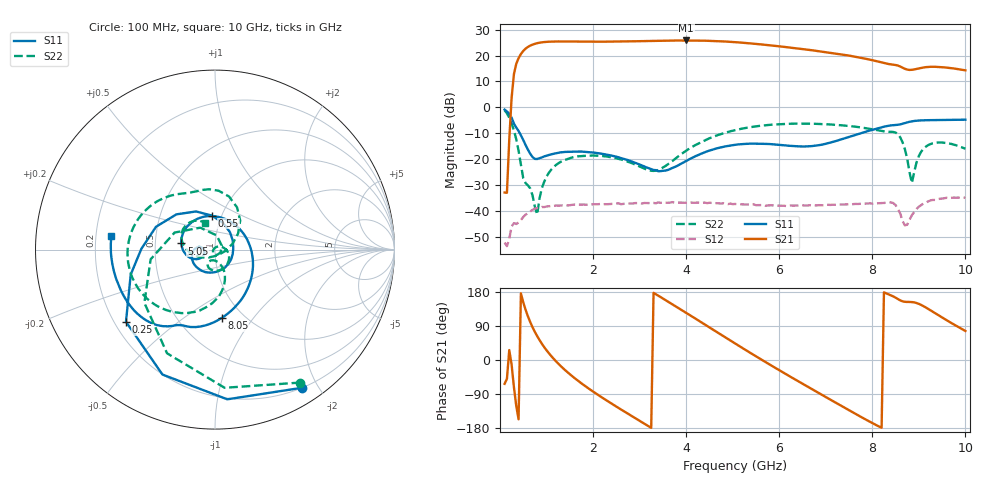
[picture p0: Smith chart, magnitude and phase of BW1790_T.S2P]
!Keysight Technologies,N5245A,MY52451660,A.10.49.11
!Date: Monday, August 07, 2017 16:27:22
!Correction: S11(Full 2 Port(1,2))
!S21(Full 2 Port(1,2))
!S12(Full 2 Port(1,2))
!S22(Full 2 Port(1,2))
!S2P File: Measurements: S11, S21, S12, S22:
# Hz S  dB  R 50
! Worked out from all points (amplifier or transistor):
!   199 points, 100 MHz to 10 GHz, reference 50 ohm
!   highest |S21| = 25.8 dB at 4 GHz (marker M1)
!   |S21| within 3 dB of that: 562.9 MHz to 6.354 GHz (5.791 GHz wide, 167 % of centre)
!   unconditionally stable (mu >= 1): start of sweep to end of sweep
!   at 1.75 GHz: K = 2.08, MAG = 25.5 dB, |S12| = -37.4 dB
!   at 5.05 GHz: K = 1.85, MAG = 25.8 dB, |S12| = -37.1 dB
!   at 10 GHz: K = 3.53, MAG = 16.1 dB, |S12| = -34.8 dB
!   S11 on the Smith chart (normalised r, x): 100 MHz: 0.20, -1.79; 250 MHz: 0.25, -0.34; 550 MHz: 0.90, +0.35; 5.05 GHz: 0.68, +0.05; 8.05 GHz: 0.80, -0.71; 10 GHz: 0.27, +0.06
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1e8  -0.82 -57.8  -32.75 -62.9  -51.98 17.9  -1.11 -57.3
2.5e8  -3.90 -141.0  3.56 -11.9  -45.81 -12.4  -6.15 -143.0
3e8  -6.20 -163.5  12.81 -71.2  -44.54 -48.9  -8.81 -171.4
3.5e8  -7.75 179.2  16.79 -121.0  -44.85 -87.8  -12.24 157.1
4.5e8  -10.71 137.6  20.58 175.8  -43.36 -169.7  -22.00 83.1
5.5e8  -14.43 95.0  22.63 132.8  -41.27 133.9  -29.10 -28.3
7.5e8  -19.81 4.9  24.50 74.2  -38.97 76.0  -38.24 -158.8
1.05e9  -18.30 -80.9  25.32 18.0  -38.02 33.0  -25.18 6.2
1.35e9  -17.22 -118.4  25.41 -21.2  -37.67 7.9  -20.53 -33.9
1.75e9  -16.98 -148.4  25.34 -61.6  -37.42 -14.0  -18.73 -69.5
2.45e9  -18.74 179.9  25.36 -119.1  -37.07 -47.2  -19.34 -108.6
2.95e9  -21.59 170.5  25.51 -156.7  -36.81 -66.4  -22.37 -117.5
3.4e9  -24.56 -175.4  25.67 169.9  -36.55 -83.9  -24.08 -86.7
4e9  -20.61 -149.6  25.80 124.5  -36.69 -109.5  -16.65 -68.3
4.5e9  -16.61 -162.4  25.65 86.1  -36.69 -127.8  -11.86 -84.3
5.05e9  -14.38 169.6  25.14 43.7  -37.14 -147.6  -8.71 -108.5
5.75e9  -14.04 123.2  24.02 -8.7  -37.72 -169.7  -6.76 -140.2
6.7e9  -14.87 33.3  22.04 -76.7  -37.72 163.3  -6.25 -179.4
7.45e9  -11.62 -40.9  20.11 -129.1  -37.30 138.4  -7.04 150.6
8.05e9  -8.35 -84.3  18.00 -169.7  -36.87 115.7  -8.55 124.3
8.35e9  -7.04 -104.0  16.72 173.4  -36.63 98.7  -9.35 107.3
1e10  -4.70 172.6  14.29 76.6  -34.77 58.6  -15.89 110.9
